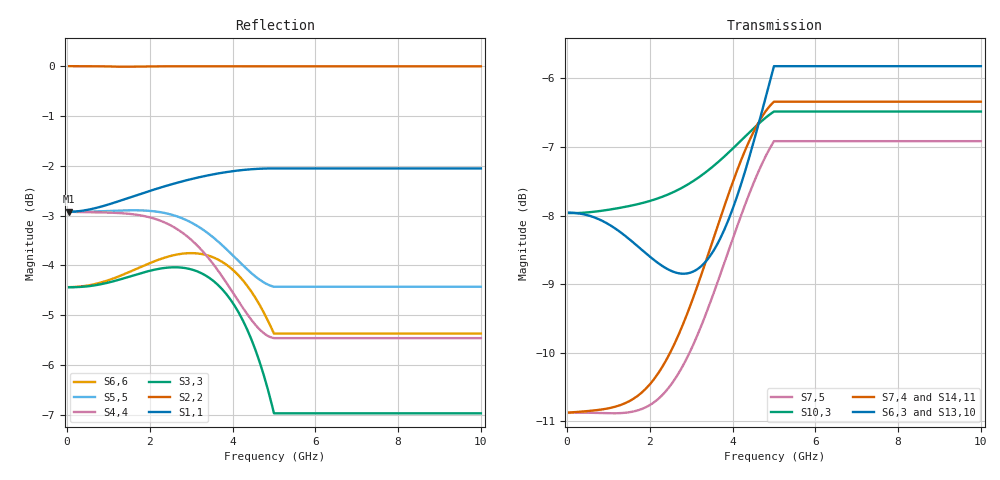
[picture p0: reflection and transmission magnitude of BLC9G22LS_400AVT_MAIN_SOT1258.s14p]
! Created Tue Apr 19 12:43:59 2016
! 14 Port Network Data from SP1.SP block
! freq  magS1_1  angS1_1  magS1_2  angS1_2  magS1_3  angS1_3  magS1_4  angS1_4
!  magS1_5  angS1_5  magS1_6  angS1_6  magS1_7  angS1_7  magS1_8  angS1_8
!  magS1_9  angS1_9  magS1_10  angS1_10  magS1_11  angS1_11  magS1_12  angS1_12
!  magS1_13  angS1_13  magS1_14  angS1_14
!  magS2_1  angS2_1  magS2_2  angS2_2
!  magS2_3  angS2_3  magS2_4  angS2_4  magS2_5  angS2_5  magS2_6  angS2_6
!  magS2_7  angS2_7  magS2_8  angS2_8  magS2_9  angS2_9  magS2_10  angS2_10
!  magS2_11  angS2_11  magS2_12  angS2_12  magS2_13  angS2_13  magS2_14  angS2_14
!  magS3_1  angS3_1  magS3_2  angS3_2  magS3_3  angS3_3  magS3_4  angS3_4
!  magS3_5  angS3_5  magS3_6  angS3_6  magS3_7  angS3_7  magS3_8  angS3_8
!  magS3_9  angS3_9  magS3_10  angS3_10  magS3_11  angS3_11  magS3_12  angS3_12
!  magS3_13  angS3_13  magS3_14  angS3_14
!  magS4_1  angS4_1  magS4_2  angS4_2
!  magS4_3  angS4_3  magS4_4  angS4_4  magS4_5  angS4_5  magS4_6  angS4_6
!  magS4_7  angS4_7  magS4_8  angS4_8  magS4_9  angS4_9  magS4_10  angS4_10
!  magS4_11  angS4_11  magS4_12  angS4_12  magS4_13  angS4_13  magS4_14  angS4_14
!  magS5_1  angS5_1  magS5_2  angS5_2  magS5_3  angS5_3  magS5_4  angS5_4
!  magS5_5  angS5_5  magS5_6  angS5_6  magS5_7  angS5_7  magS5_8  angS5_8
!  magS5_9  angS5_9  magS5_10  angS5_10  magS5_11  angS5_11  magS5_12  angS5_12
!  magS5_13  angS5_13  magS5_14  angS5_14
!  magS6_1  angS6_1  magS6_2  angS6_2
!  magS6_3  angS6_3  magS6_4  angS6_4  magS6_5  angS6_5  magS6_6  angS6_6
!  magS6_7  angS6_7  magS6_8  angS6_8  magS6_9  angS6_9  magS6_10  angS6_10
!  magS6_11  angS6_11  magS6_12  angS6_12  magS6_13  angS6_13  magS6_14  angS6_14
!  magS7_1  angS7_1  magS7_2  angS7_2  magS7_3  angS7_3  magS7_4  angS7_4
!  magS7_5  angS7_5  magS7_6  angS7_6  magS7_7  angS7_7  magS7_8  angS7_8
!  magS7_9  angS7_9  magS7_10  angS7_10  magS7_11  angS7_11  magS7_12  angS7_12
!  magS7_13  angS7_13  magS7_14  angS7_14
!  magS8_1  angS8_1  magS8_2  angS8_2
!  magS8_3  angS8_3  magS8_4  angS8_4  magS8_5  angS8_5  magS8_6  angS8_6
!  magS8_7  angS8_7  magS8_8  angS8_8  magS8_9  angS8_9  magS8_10  angS8_10
!  magS8_11  angS8_11  magS8_12  angS8_12  magS8_13  angS8_13  magS8_14  angS8_14
!  magS9_1  angS9_1  magS9_2  angS9_2  magS9_3  angS9_3  magS9_4  angS9_4
!  magS9_5  angS9_5  magS9_6  angS9_6  magS9_7  angS9_7  magS9_8  angS9_8
!  magS9_9  angS9_9  magS9_10  angS9_10  magS9_11  angS9_11  magS9_12  angS9_12
!  magS9_13  angS9_13  magS9_14  angS9_14
!  magS10_1  angS10_1  magS10_2  angS10_2
!  magS10_3  angS10_3  magS10_4  angS10_4  magS10_5  angS10_5  magS10_6  angS10_6
!  magS10_7  angS10_7  magS10_8  angS10_8  magS10_9  angS10_9  magS10_10  angS10_10
!  magS10_11  angS10_11  magS10_12  angS10_12  magS10_13  angS10_13  magS10_14  angS10_14
!  magS11_1  angS11_1  magS11_2  angS11_2  magS11_3  angS11_3  magS11_4  angS11_4
!  magS11_5  angS11_5  magS11_6  angS11_6  magS11_7  angS11_7  magS11_8  angS11_8
!  magS11_9  angS11_9  magS11_10  angS11_10  magS11_11  angS11_11  magS11_12  angS11_12
!  magS11_13  angS11_13  magS11_14  angS11_14
!  magS12_1  angS12_1  magS12_2  angS12_2
!  magS12_3  angS12_3  magS12_4  angS12_4  magS12_5  angS12_5  magS12_6  angS12_6
!  magS12_7  angS12_7  magS12_8  angS12_8  magS12_9  angS12_9  magS12_10  angS12_10
!  magS12_11  angS12_11  magS12_12  angS12_12  magS12_13  angS12_13  magS12_14  angS12_14
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# ghz S ma R 50
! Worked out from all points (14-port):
!   200 points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, 50 MHz to 10 GHz, reference 50 ohm
!   strongest paths, dB at 50 MHz, 2.55 GHz, 5.05 GHz, 7.55 GHz, 10 GHz:
!     S6,3: -8.0, -8.8, -5.8, -5.8, -5.8
!     S13,10: -8.0, -8.8, -5.9, -5.9, -5.9
!     S7,4: -10.9, -9.9, -6.3, -6.3, -6.3
!     S14,11: -10.9, -9.9, -6.4, -6.4, -6.4
!     S10,3: -8.0, -7.7, -6.5, -6.5, -6.5
!     S7,5: -10.9, -10.4, -6.9, -6.9, -6.9
!   lowest |S11| = -2.9 dB at 50 MHz (marker M1), VSWR 6.00, Z = 8.34 + j0.00314 ohm
!   |S11| at or under -10 dB: nowhere
